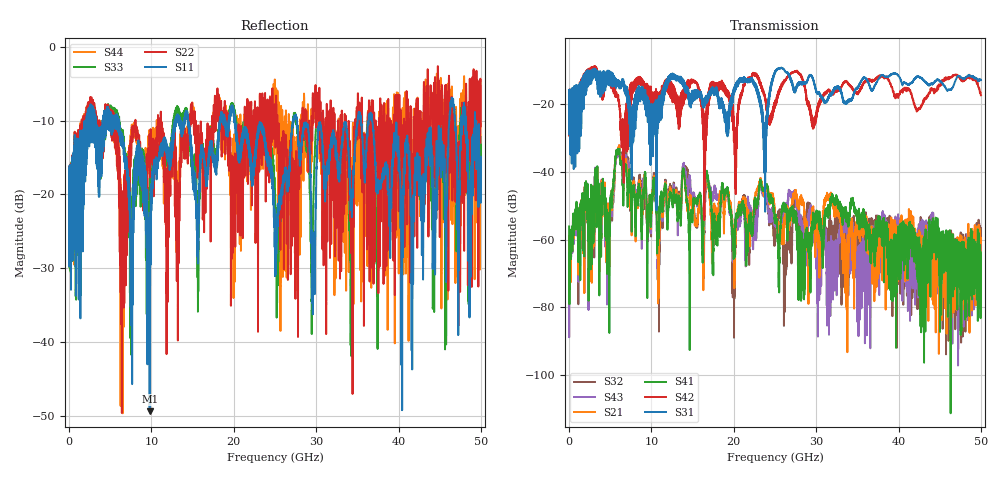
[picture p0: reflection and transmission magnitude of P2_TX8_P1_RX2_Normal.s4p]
!Keysight Technologies,N5225B,MY57041031,A.13.20.10
!Date: Friday, May 31, 2019 11:16:58
!Correction: S11(Full 4 Port(1,2,3,4))
!S12(Full 4 Port(1,2,3,4))
!S13(Full 4 Port(1,2,3,4))
!S14(Full 4 Port(1,2,3,4))
!S21(Full 4 Port(1,2,3,4))
!S22(Full 4 Port(1,2,3,4))
!S23(Full 4 Port(1,2,3,4))
!S24(Full 4 Port(1,2,3,4))
!S31(Full 4 Port(1,2,3,4))
!S32(Full 4 Port(1,2,3,4))
!S33(Full 4 Port(1,2,3,4))
!S34(Full 4 Port(1,2,3,4))
!S41(Full 4 Port(1,2,3,4))
!S42(Full 4 Port(1,2,3,4))
!S43(Full 4 Port(1,2,3,4))
!S44(Full 4 Port(1,2,3,4))
!S4P File: Measurements: <S11,S12,S13,S14>,
!<S21,S22,S23,S24>,
!<S31,S32,S33,S34>,
!<S41,S42,S43,S44>:
# Hz S  dB  R 50.0
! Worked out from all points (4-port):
!   5000 points, 10 MHz to 50 GHz, reference 50 ohm
!   strongest paths, dB at 10 MHz, 12.51 GHz, 25.01 GHz, 37.51 GHz, 50 GHz:
!     S31: -19.3, -11.5, -10.3, -12.8, -12.8
!     S42: -19.5, -16.2, -19.4, -11.8, -17.3
!     S41: -56.1, -47.6, -54.4, -55.5, -73.1
!     S21: -67.7, -47.4, -53.0, -64.6, -60.8
!     S43: -66.1, -46.9, -53.6, -56.0, -71.4
!     S32: -58.9, -46.5, -57.7, -54.2, -61.7
!   lowest |S11| = -49.4 dB at 9.79 GHz (marker M1), VSWR 1.01, Z = 49.8 - j0.288 ohm
!   |S11| at or under -10 dB: 20.17 GHz to 27.19 GHz (7.015 GHz wide, 29.6 % of centre); 27.67 GHz to 35.04 GHz (7.369 GHz wide, 23.5 % of centre); 36.79 GHz to 46.17 GHz (9.379 GHz wide, 22.6 % of centre)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
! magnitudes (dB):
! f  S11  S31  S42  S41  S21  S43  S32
! 10 MHz  -19.6  -19.3  -19.5  -56.1  -67.7  -66.1  -58.9
! 3.38 GHz  -16.2  -13.1  -11.3  -42.3  -42.6  -40.9  -41.4
! 4.76 GHz  -8.4  -10.5  -11.7  -68.3  -60.7  -69.2  -60.8
! 5.95 GHz  -11.5  -14.1  -18.0  -33.1  -32.7  -33.6  -33.1
! 9.79 GHz  -49.4  -26.0  -17.2  -46.8  -47.2  -46.9  -46.8
! 14.2 GHz  -8.7  -16.1  -15.8  -46.2  -47.2  -41.4  -39.2
! 50 GHz  -14.9  -12.8  -17.3  -73.1  -60.8  -71.4  -61.7
